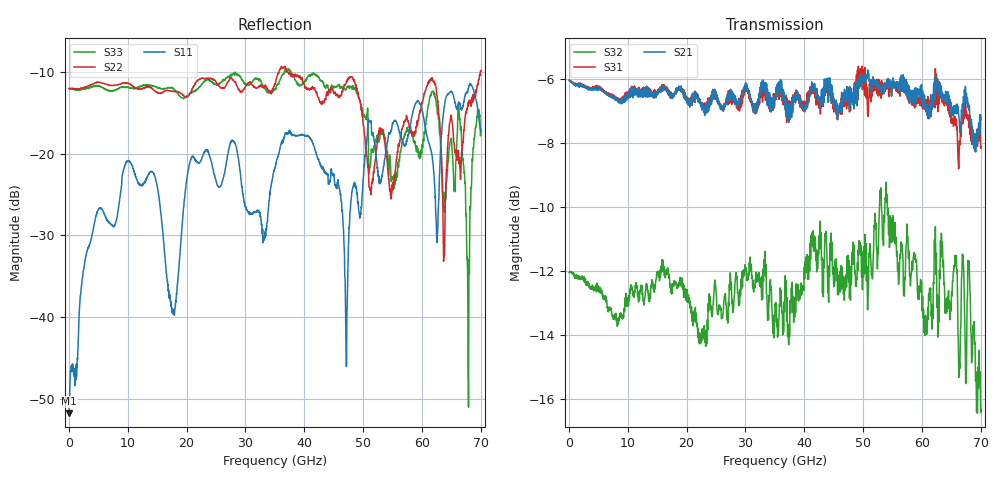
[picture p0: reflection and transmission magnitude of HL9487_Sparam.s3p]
! 10/4/2022 8:51:13 AM
! H:\PRODUCTION_DATA\TEMP_S3P.S3P
! CHANNEL.1
! TR.MEASUREMENT
! CORRECTED.DATA
# GHZ S RI R 50.0
! FREQ.GHZ  S11RE  S11IM  S12RE  S12IM  S13RE  S13IM
!  S21RE  S21IM  S22RE  S22IM  S23RE  S23IM
!  S31RE  S31IM  S32RE  S32IM  S33RE  S33IM
!; PortSelection: Port_123
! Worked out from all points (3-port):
!   2000 points, 35 MHz to 70 GHz, reference 50 ohm
!   strongest paths, dB at 35 MHz, 17.54 GHz, 35.03 GHz, 52.53 GHz, 70 GHz:
!     S21: -6.1, -6.6, -6.5, -6.3, -7.3
!     S31: -6.0, -6.5, -6.6, -6.3, -8.1
!     S32: -12.1, -12.4, -13.0, -11.5, -16.3
!   lowest |S11| = -51.8 dB at 35 MHz (marker M1), VSWR 1.01, Z = 50.2 + j0.0646 ohm
!   |S11| at or under -10 dB: start of sweep to end of sweep
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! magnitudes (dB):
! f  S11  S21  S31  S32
! 35 MHz  -51.8  -6.1  -6.0  -12.1
! 9.87 GHz  -20.9  -6.5  -6.4  -12.8
! 17.71 GHz  -39.7  -6.5  -6.5  -12.4
! 20.89 GHz  -20.4  -6.8  -6.8  -13.6
! 35.03 GHz  -21.7  -6.5  -6.6  -13.0
! 47.15 GHz  -46.1  -6.5  -6.7  -12.5
! 51.03 GHz  -16.1  -6.1  -6.4  -11.6
! 66.36 GHz  -13.9  -7.5  -7.9  -14.9
! 67.8 GHz  -12.2  -6.9  -7.3  -11.7
! 70 GHz  -17.3  -7.3  -8.1  -16.3
